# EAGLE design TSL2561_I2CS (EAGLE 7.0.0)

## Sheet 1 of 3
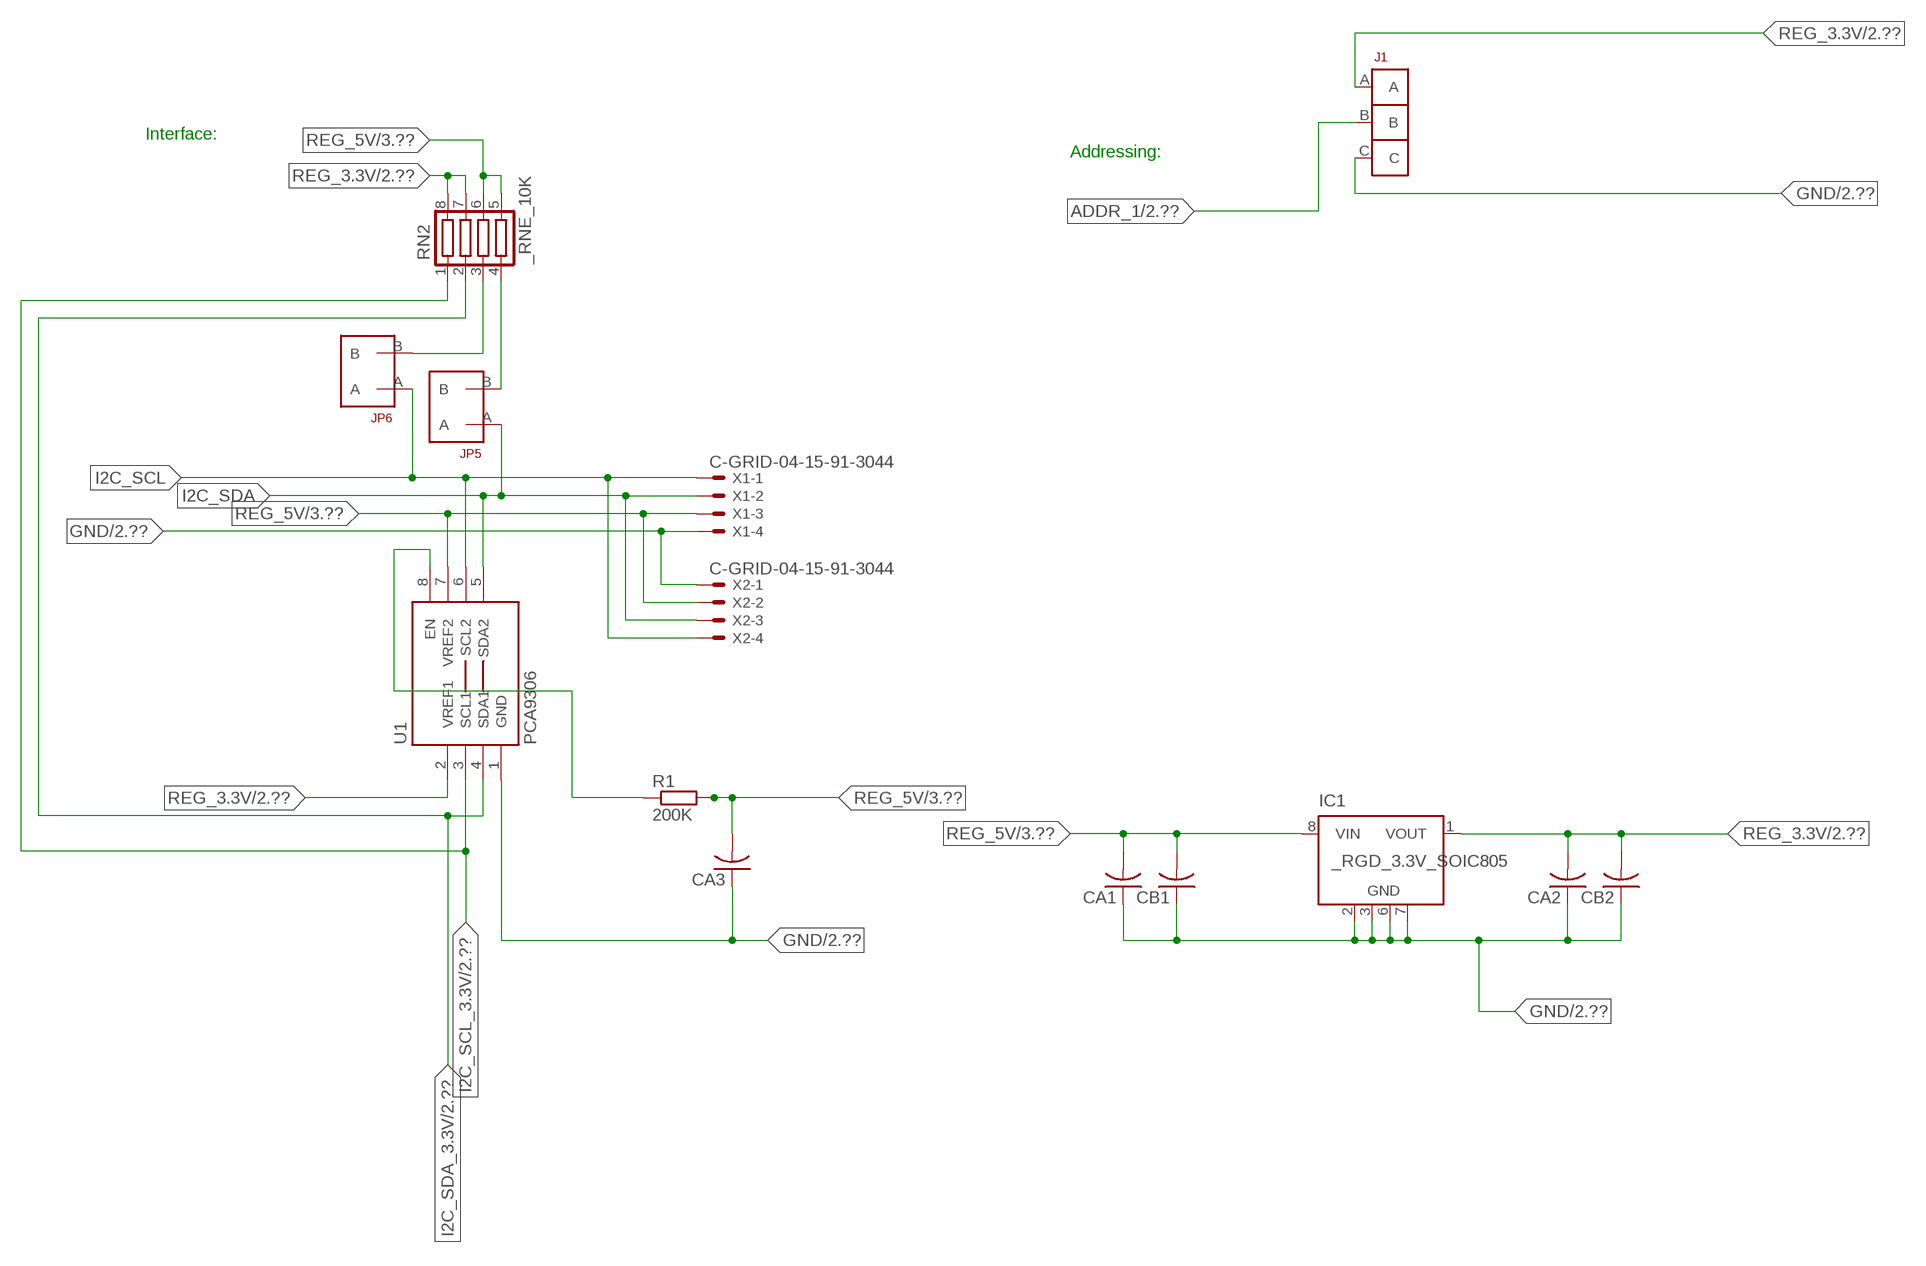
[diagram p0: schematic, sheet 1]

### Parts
CA1  CC1206KRX7R9BB104  [.1UF]
CA2  CC1206KRX7R9BB104  [.1UF]
CA3  CC1206KRX7R9BB104  [.1UF]
CB1  TMK316F106ZL-TC1206K  [TMK316F106ZL-T]
CB2  TMK316F106ZL-TC1206K  [TMK316F106ZL-T]
IC1  _RGD_3.3V_SOIC805  [_RGC_3.3V_SOIC8]
J1  JUMPER_1X3_2MM  [JUMPER_1X3_2MM]
JP5  JUMPER_1X2_2MM  [JUMPER_1X2_2MM]
JP6  JUMPER_1X2_2MM  [JUMPER_1X2_2MM]
R1  200K  RESISTOR_SMT-0603  [R603]
RN2  _RNE_10K  [RNE]
U1  PCA9306  PCA9306_NCD  [PSOP-8]
X1  C-GRID-04-15-91-3044  [15-91-04]
X2  C-GRID-04-15-91-3044  [15-91-04]

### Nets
ADDR_1: J1.B ; also sheet 2
GND: CA1.1 CA2.1 CA3.1 CB1.1 CB2.1 IC1.2(GND) IC1.3(GND) IC1.6(GND) IC1.7(GND) J1.C U1.1(GND) X1.4 X2.1 ; also sheet 2,3
I2C_SCL: JP6.A U1.6(SCL2) X1.1 X2.4
I2C_SCL_3.3V: RN2.1 U1.3(SCL1) ; also sheet 2
I2C_SDA: JP5.A U1.5(SDA2) X1.2 X2.3
I2C_SDA_3.3V: RN2.2 U1.4(SDA1) ; also sheet 2
N$1: JP6.B RN2.3
N$2: JP5.B RN2.4
N$23: R1.1 U1.8(EN)
REG_3.3V: CA2.2 CB2.2 IC1.1(VOUT) J1.A RN2.7 RN2.8 U1.2(VREF1) ; also sheet 2
REG_5V: CA1.2 CA3.2 CB1.2 IC1.8(VIN) R1.2 RN2.5 RN2.6 U1.7(VREF2) X1.3 X2.2 ; also sheet 3
Unconnected: IC1.4(NC) IC1.5(NC)

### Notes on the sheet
- Interface:
- Addressing:

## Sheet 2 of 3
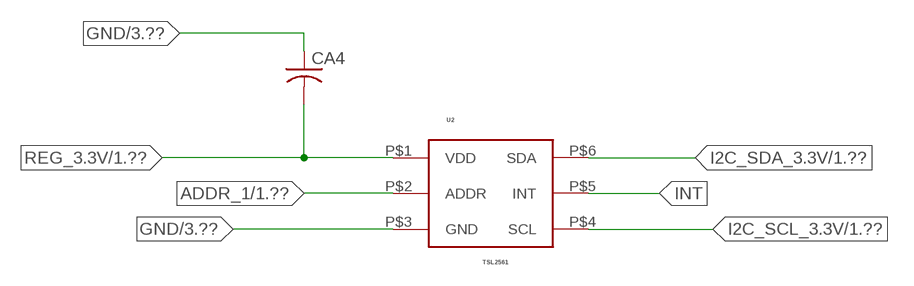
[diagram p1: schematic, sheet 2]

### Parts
CA4  _CA_.10UF_50VC1206K  [_CA_.1UF_50V]
U2  TSL2561  [TSL2561]

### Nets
ADDR_1: U2.P$2(ADDR) ; also sheet 1
GND: CA4.1 U2.P$3(GND) ; also sheet 1,3
I2C_SCL_3.3V: U2.P$4(SCL) ; also sheet 1
I2C_SDA_3.3V: U2.P$6(SDA) ; also sheet 1
INT: U2.P$5(INT)
REG_3.3V: CA4.2 U2.P$1(VDD) ; also sheet 1

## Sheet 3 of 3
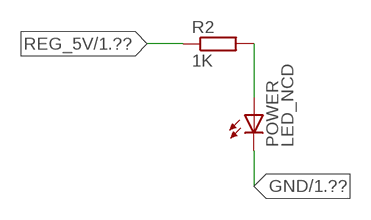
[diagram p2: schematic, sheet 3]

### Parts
POWER  LED_NCD  [CHIPLED_0603]
R2  1K  RESISTOR_SMT-0402  [R402]

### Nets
GND: POWER.C ; also sheet 1,2
N$4: POWER.A R2.2
REG_5V: R2.1 ; also sheet 1

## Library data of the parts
CA1-CA3 = NCD_ULTIMATE_LIBRARY:CC1206KRX7R9BB104: Capacitor CA .1uF 50V SMT C1206K CC1206KRX7R9BB104
CA4 = NCD_ULTIMATE_LIBRARY:_CA_.10UF_50V: Capacitor .1uF SMT
CB1 CB2 = NCD_ULTIMATE_LIBRARY:TMK316F106ZL-T: Capacitor CB 10uF SMT 1206 TMK316F106ZL-T
IC1 = NCD_ULTIMATE_LIBRARY:_RGD_3.3V_SOIC8: Regulator Linear 3.3V Chip Positive VOLTAGE REGULATOR Digikey 497-1199-2-ND/L78L33ACD13TR
J1 = NCD_ULTIMATE_CONNECTORS:JUMPER_1X3_2MM
JP5 JP6 = NCD_ULTIMATE_CONNECTORS:JUMPER_1X2_2MM
POWER = NCD_ULTIMATE_LIBRARY:LED_NCD: LED Digikey 754-1132-2-ND/APT2012SRCPRV
R1 R2 = NCD_ULTIMATE_LIBRARY:RESISTOR_SMT: NCD Resistor
RN2 = NCD_ULTIMATE_LIBRARY:_RNE_10K: Resistor Array RNE SMT 10K x 4 Single Resistor Source: http://www.ctscorp.com/components/Datasheets/CTSChipArrayDs.pdf Digikey 742C083103JPTR-ND/742C083103JP; OC_FARNELL: unknown; OC_NEWARK: unknown
U1 = NCD_ULTIMATE_LIBRARY:PCA9306_NCD: NCD Bidirectional I2C level shifter. NOT compatible with all available part number pinout schemes- DOUBLE CHECK!!!; PROD_ID: IC-10023
U2 = NCD_ULTIMATE_bhaskar:TSL2561
X1 X2 = NCD_ULTIMATE_CONNECTORS:C-GRID-04: CONNECTOR 4-Pos I2C wire to board 2.54 mm (0.100") pitch header Digikey WM1342-ND/0015912045; OC_FARNELL: unknown; OC_NEWARK: unknown

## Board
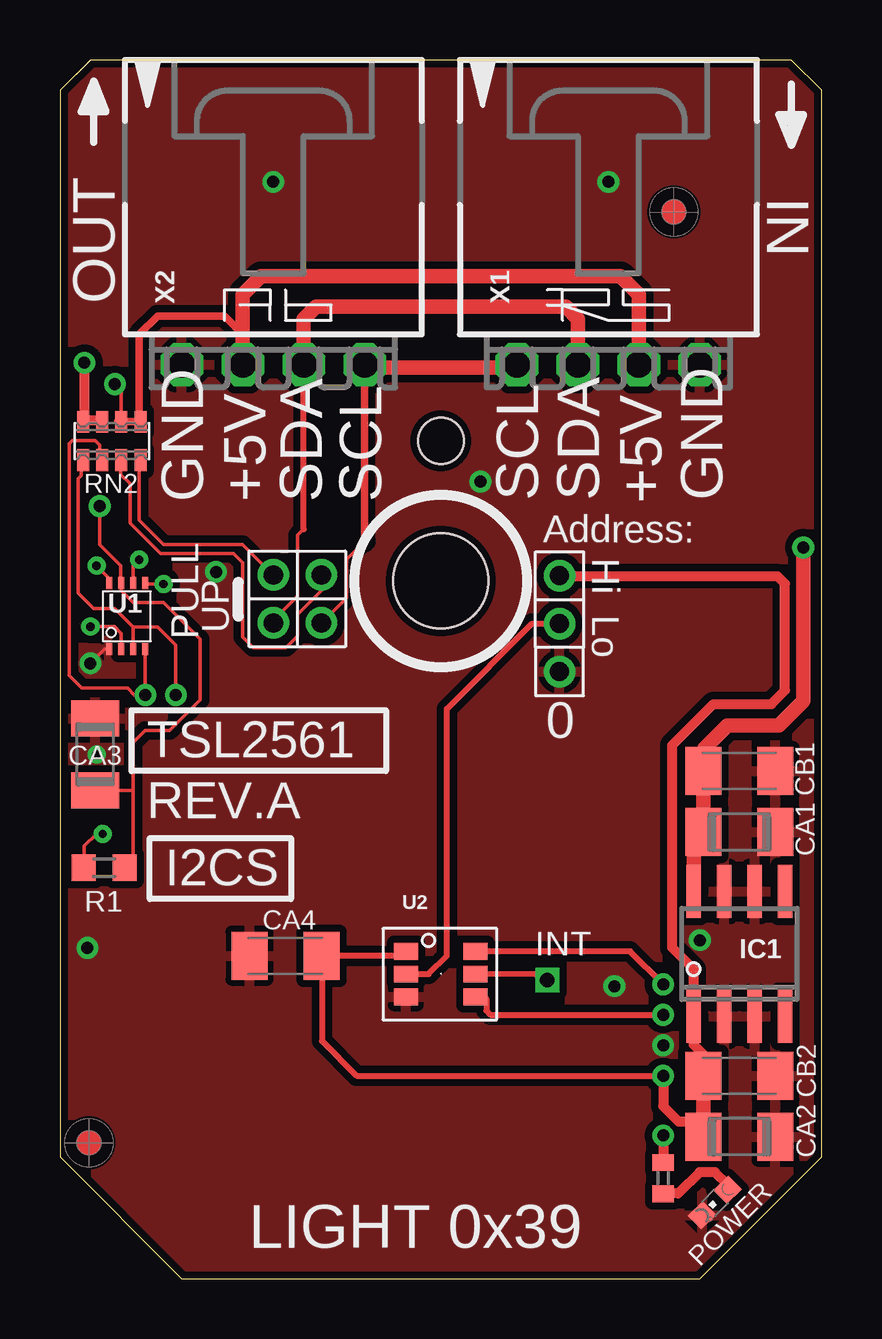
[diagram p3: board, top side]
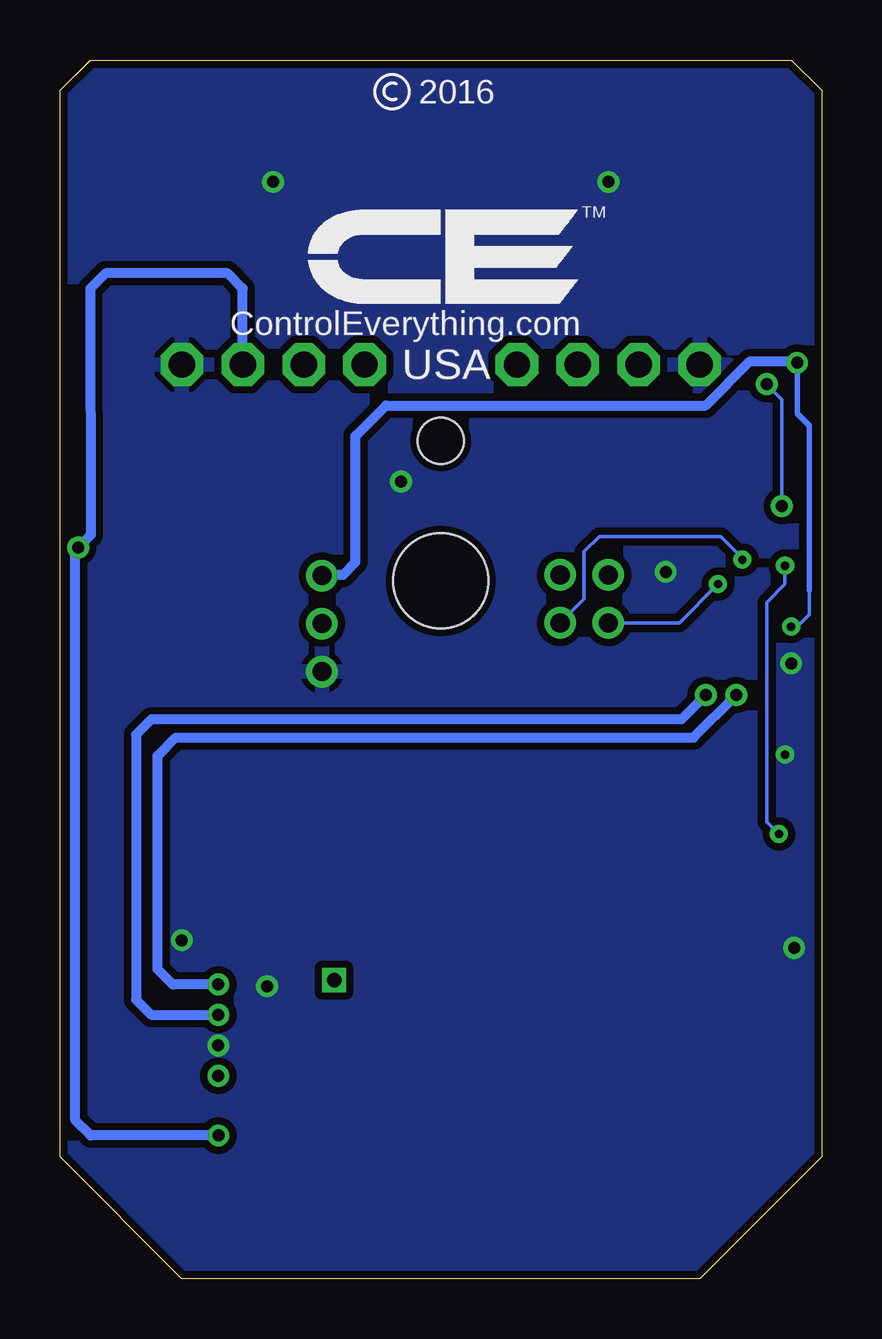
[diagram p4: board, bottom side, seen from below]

Size 31.75 x 50.8 mm. Coordinates in mm from the lower left corner, seen from the top.
Outline: 48 segments
Copper layers (1*16): Top 0.035mm / dielectric 1.5mm / Bottom 0.035mm
Design rules "default": minimum track width 5mil, minimum drill 24mil, track to track 5mil, track to pad 5mil, pad to pad 5mil, via to via 5mil, smd to smd 5mil, copper to edge 10mil, drill to drill 8mil, minimum pad ring 10mil, minimum via ring 8mil, stop-mask expansion 2mil, vias tented up to drill 0mil, thermal gap 10mil
Holes 3.96 mm at 15.88,29.08
Holes 1.91 mm at 15.88,34.93

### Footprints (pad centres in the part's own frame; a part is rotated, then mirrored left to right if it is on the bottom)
.1UF = smd 1.5 x 2: 1 -1.5,0; 2 1.5,0
_CA_.1UF_50V = smd 1.5 x 2: 1 -1.5,0; 2 1.5,0
TMK316F106ZL-T = smd 1.5 x 2: 1 -1.5,0; 2 1.5,0
_RGC_3.3V_SOIC8 = smd 0.6 x 2.2: 1 -1.905,-2.6; 2 -0.635,-2.6; 3 0.635,-2.6; 4 1.905,-2.6; 5 1.905,2.6; 6 0.635,2.6; 7 -0.635,2.6; 8 -1.905,2.6
JUMPER_1X3_2MM = drill 0.8: A 0,2; B 0,0; C 0,-2
JUMPER_1X2_2MM = drill 0.8: A 0,2; B 0,0
CHIPLED_0603 = smd 0.8 x 0.876: A 0,-0.75; C 0,0.75
R603 = smd 1 x 1.1: 1 -0.85,0; 2 0.85,0
R402 = smd 0.7 x 0.9: 1 -0.65,0; 2 0.65,0
RNE = smd 0.5 x 0.9: 1 -1.2,-0.8; 2 -0.4,-0.8; 3 0.4,-0.8; 4 1.2,-0.8; 5 1.2,0.8; 6 0.4,0.8; 7 -0.4,0.8; 8 -1.2,0.8
PSOP-8 = smd 0.25 x 0.5: 1 -0.73,-1.37; 2 -0.23,-1.37; 3 0.27,-1.37; 4 0.77,-1.37; 5 0.77,1.38; 6 0.27,1.38; 7 -0.23,1.38; 8 -0.73,1.38
TSL2561 = smd 1 x 0.7: P$1 -0.95,0.95; P$2 -0.95,0; P$3 -0.95,-0.95; P$4 1.95,-0.95; P$5 1.95,0; P$6 1.95,0.95
15-91-04 = drill 1.1 pad 1.778 octagon: 1 -3.81,-7.62; 2 -1.27,-7.62; 3 1.27,-7.62; 4 3.81,-7.62

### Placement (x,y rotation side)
CA1  28.32,18.62 180 top
CA2  28.32,5.92 180 top
CA3  1.46,21.86 270 top
CA4  9.4,13.46 0 top
CB1  28.32,21.16 180 top
CB2  28.32,8.46 180 top
IC1  28.32,13.54 0 top
J1  20.83,27.31 0 top
JP5  8.89,29.34 180 top
JP6  10.9,29.34 180 top
POWER  27.3,3.18 135 top
R1  1.84,17.13 0 top
R2  25.15,4.19 270 top
RN2  2.16,34.93 0 top
U1  2.79,27.61 0 top
U2  15.37,12.7 0 top
U$5  [VISION_REF10]  1.21,5.66 90 top
U$28  [VISION_REF10]  25.59,44.46 90 top
X1  22.86,45.72 0 top
X2  8.89,45.72 0 top

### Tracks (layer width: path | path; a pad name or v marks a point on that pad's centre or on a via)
ADDR_1
  Top 0.254: U2.P$2 15.37,12.7 16.13,13.46 16.13,23.75 19.68,27.31 J1.B
GND  (via drill 0.35, 0.5)
  Top 0.152: CA3.1 1.52,23.42 1.52,23.62 | v1.27,25.65 1.86,26.24 U1.1
  other vias: 8.89,45.72 22.86,45.72 25.15,9.73 17.53,33.22 26.67,14.11 1.15,13.79 6.5,29.46 23.11,12.19 1.52,21.84
  pour Top (isolate 0.305): -1.27,0 -1.27,50.8 33.02,50.8 33.02,0
  pour Bottom (isolate 0.305): -5.08,0 -5.08,50.8 35.56,50.8 35.56,0
I2C_SCL  (via drill 0.35)
  Top 0.152: 12.7,30.73 11.94,29.97 11.94,28.38 JP6.A | v3.3,29.97 3.06,29.73 U1.6
  Top 0.305: 12.7,30.73 X2.4
  Top 0.406: X2.4 12.7,37.97 | 19.05,37.97 X1.1
  Top 0.61: 12.7,37.97 19.05,37.97
  Bottom 0.152: JP6.A 9.91,28.33 9.91,30.3 9.27,30.94 4.19,30.94 3.3,30.05 v3.3,29.97
I2C_SCL_3.3V  (via drill 0.5)
  Top 0.152: RN2.1 0.89,34.07 0.89,33.48 0.77,33.35 0.77,28.59 1.41,27.94 2.29,27.94 3.06,27.17 | 3.06,27.17 U1.3 | v4.83,24.33 v4.83,24.34 4.83,26.42 4.08,27.17 3.06,27.17
  Top 0.254: U2.P$4 17.78,11.67 17.78,11.18 17.96,11 v25.15,11
  Bottom 0.406: v4.83,24.33 5.84,23.32 27.94,23.32 28.58,22.68 28.58,11.63 27.94,11 v25.15,11
I2C_SDA  (via drill 0.35)
  Top 0.152: JP5.A 8.89,27.44 9.91,28.45 9.91,30.99 10.16,31.24 | U1.5 3.6,28.96 v4.32,28.96
  Top 0.254: 10.16,31.24 10.16,31.25 X2.3
  Top 0.61: X2.3 10.16,40.01 10.67,40.51 21.09,40.51 21.59,40.01 X1.2
  Bottom 0.152: v4.32,28.96 5.94,27.34 JP5.A
I2C_SDA_3.3V  (via drill 0.5)
  Top 0.152: RN2.2 1.65,34.14 1.65,34.75 1.46,34.94 0.51,34.94 0.38,34.81 0.38,26.37 0.38,26.36 0.38,25.15 0.91,24.61 2.82,24.61 3.1,24.33 v3.56,24.33 v3.56,24.34 U1.4
  Top 0.254: v25.15,12.27 23.77,13.65 U2.P$6
  Bottom 0.406: v25.15,12.27 27.05,12.27 27.69,12.9 27.69,21.79 26.93,22.56 5.34,22.56 v3.56,24.33
INT  (via drill 0.6)
  Top 0.229: U2.P$5 19.81,12.7 20.07,12.45 v20.32,12.45
N$1
  Top 0.152: JP6.B 10.92,29.31 10.92,28.7 9.91,27.69 9.91,26.8 9.42,26.31 8.06,26.31 7.62,26.75 7.62,29.84 7.24,30.23 4.19,30.23 2.92,31.5 2.92,33.15 2.54,33.53 2.54,34.1 RN2.3
  Top 0.305: 2.54,34.02 RN2.3
N$2
  Top 0.152: JP5.B 7.62,30.61 4.32,30.61 3.3,31.62 3.3,34.07 RN2.4
  Top 0.305: 3.37,33.88 RN2.4
N$4
  Top 0.406: POWER.A 27.84,3.92 27.3,4.45 26.67,4.45 25.78,3.56 25.16,3.56 R2.2
N$23  (via drill 0.35)
  Top 0.152: R1.1 1.02,17.16 1.02,18.03 1.52,18.54 v1.78,18.54 | v1.52,29.72 2.06,29.18 U1.8
  Bottom 0.152: v1.78,18.54 2.29,19.05 2.29,28.19 1.52,28.96 v1.52,29.72
REG_3.3V  (via drill 0.35, 0.5)
  Top 0.152: v1.27,27.18 2.29,27.18 2.56,26.9 U1.2
  Top 0.254: v25.15,8.46 12.37,8.46 10.92,9.91 10.92,13.44 CA4.2 14.61,13.46 U2.P$1
  Top 0.406: CB2.2 26.82,9.35 26.42,9.75 26.42,10.36 | v25.15,8.46 25.15,7.19 25.78,6.55 26.82,6.55 | IC1.1 26.42,12.9 25.53,13.79 25.53,22.24 27.24,23.95 29.66,23.95 30.23,24.52 30.23,28.97 29.91,29.29 20.85,29.29 J1.A | 26.52,5.62 CA2.2 | v1.02,38.18 1.02,35.78 | 1.02,35.78 RN2.8 | 1.02,35.78 1.71,35.78 RN2.7
  Top 0.61: CB2.2 26.82,6.55 CA2.2 | 26.42,10.36 IC1.1
  Bottom 0.152: 0.51,28.7 0.51,27.69 1.02,27.18 v1.27,27.18
  Bottom 0.229: 0.51,28.7 0.51,35.56 1.02,36.07 v1.02,38.18
  Bottom 0.406: v1.02,38.18 1.08,38.24 2.99,38.24 4.83,36.4 18.16,36.4 19.43,35.13 19.43,29.87 19.94,29.34 20.83,29.34 J1.A
REG_5V  (via drill 0.5)
  Top 0.152: RN2.6 2.56,37.01 v2.29,37.29 | R1.2 3.05,17.49 3.05,20.36 | 3.05,20.36 3.05,22.35 3.56,22.86 4.57,22.86 5.84,24.13 5.84,26.67 4.32,28.19 3.05,28.19 2.56,28.68 U1.7 2.54,29.01 2.54,29.72 1.65,30.6 v1.65,32.21 | CA3.2 3.05,20.36
  Top 0.305: 7.62,39.37 7.5,39.37 | 2.42,35.74 RN2.6 RN2.5 3.31,35.8 3.31,39.37 4.07,40.13 6.86,40.13 7.62,39.37 | X2.2 7.62,39.37
  Top 0.406: v25.15,5.97 R2.1
  Top 0.61: X2.2 7.62,41.02 8.38,41.78 23.37,41.78 24.13,41.02 X1.3 | IC1.8 26.42,18.21 CA1.2 CB1.2 26.86,21.2 26.86,22.11 27.82,23.06 29.98,23.06 30.99,24.08 v30.99,30.48
  Bottom 0.152: v1.65,32.21 1.65,36.65 v2.29,37.29
  Bottom 0.406: X1.3 24.13,41.28 24.77,41.91 29.84,41.91 30.48,41.27 30.47,31 v30.99,30.48 31.11,30.36 31.11,6.6 30.48,5.97 v25.15,5.97

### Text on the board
tNames: IN | OUT | GND | +5V | SDA | SCL | SCL | SDA | +5V | GND | Address: | Hi Lo | PULL | UP | 0 | TSL2561 | REV.A | I2CS | INT | LIGHT 0x39
bNames: 2016 | TM | ControlEverything.com | USA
